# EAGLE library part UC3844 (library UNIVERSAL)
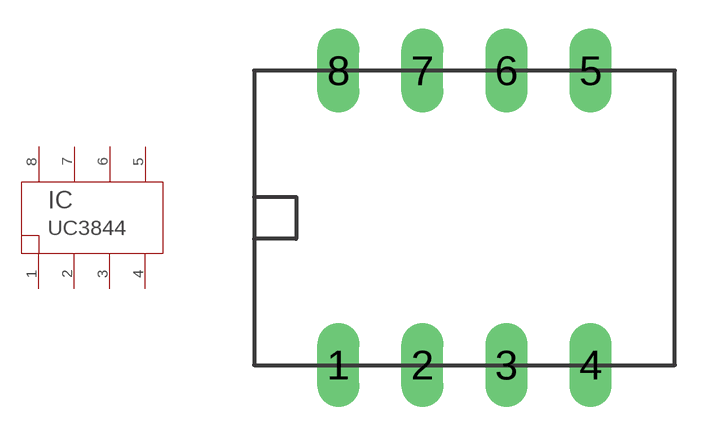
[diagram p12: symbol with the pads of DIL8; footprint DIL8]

Designator prefix IC

## UC3844  [DIL8]
1  1
2  2
3  3
4  4
5  5
6  6
7  7
8  8

## Footprint DIL8 (pad centres in mm)
drill 0.61 pad 1.27 long: 1 0,0; 2 2.54,0; 3 5.08,0; 4 7.62,0; 5 7.62,8.89; 6 5.08,8.89; 7 2.54,8.89; 8 0,8.89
